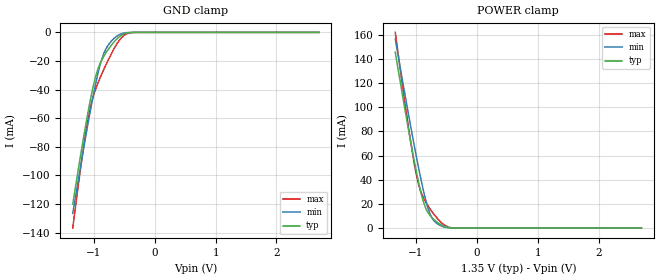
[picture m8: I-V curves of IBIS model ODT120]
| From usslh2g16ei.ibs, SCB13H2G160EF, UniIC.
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|   Model ODT120
[Model]  ODT120
Model_type Input
Vinl =   0.5750V
Vinh =   0.7750V
| variable   typ   min   max
C_comp   1.0500pF   1.0000pF   1.1000pF
| variable   typ   min   max
[Temperature Range]   45.000   95.000   -40.0000
| variable   typ   min   max
[Voltage Range]   1.35V   1.283V   1.4250V
| variable   typ   min   max
[POWER Clamp Reference] 1.35V   1.283V   1.4250V
| variable   typ   min   max
[GND Clamp Reference]   0.000V   0.000V   0.000V
[Add Submodel]
| Submodel Name   Mode
120ohm_ODT   Non-Driving
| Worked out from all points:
|   GND clamp passes 1 mA (typ) near -0.50 V on its own axis
|   POWER clamp passes 1 mA (typ) near -0.51 V on its own axis
[GND_clamp]
|Voltage   I(typ)   I(min)   I(max)
-1.35V    -120.2mA   -126.6mA   -136.9mA
-1.23V    -88.34mA   -95.9mA    -97.82mA
-1.14V    -65.66mA   -73.61mA   -71.4mA
-1.08V    -51.6mA    -59.33mA   -56.75mA
-1.02V    -39.02mA   -45.77mA   -45.84mA
-960mV    -28.85mA   -33.36mA   -38.11mA
-900mV    -21.72mA   -22.78mA   -31.76mA
-810mV    -14.7mA    -12.03mA   -23.22mA
-660mV    -6.182mA   -3.801mA   -10.58mA
-510mV    -1.116mA   -502.7uA   -2.242mA
-300mV    -9.735uA   -5.245uA   -17.77uA
2.7V      0A         0A         0A
[POWER_clamp]
|Voltage   I(typ)   I(min)   I(max)
-1.34V    145.4mA    156.2mA    161.8mA
-1.2V     103.8mA    115.9mA    110.3mA
-1.1V     75.06mA    87.82mA    75.66mA
-1.02V    53.32mA    66.13mA    51.11mA
-960mV    38.36mA    50.57mA    36.78mA
-920mV    29.52mA    40.72mA    30.13mA
-860mV    19.05mA    27.19mA    23.4mA
-780mV    11.23mA    13.2mA     16.7mA
-700mV    6.951mA    5.865mA    11.08mA
-560mV    2.052mA    1.298mA    3.566mA
-340mV    28uA       19.06uA    41.51uA
2.7V      0A         0A         0A
